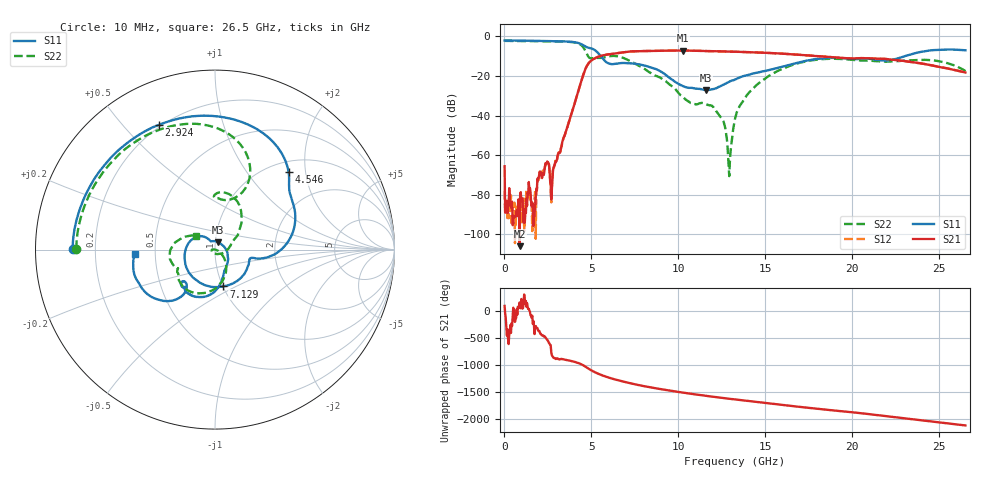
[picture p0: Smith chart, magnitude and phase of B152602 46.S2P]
!  2-Port S-parameters saved by WinCal
! VAR MeasName=S-Parameters (CALIBRATED_DATA) read from VNA (N5242A)
! VAR MeasDate=2016-1-5 16:32:47
! VAR NAME=B152602 46
! VAR FILENAME=B152602 46.S2P
! VAR DATE=2016-1-5 16:32:47
! VAR PHYS_PORTS=1,2
# Hz S DB R 50
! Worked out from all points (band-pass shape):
!   801 points, 10 MHz to 26.5 GHz, reference 50 ohm
!   highest |S21| = -7.09 dB at 10.27 GHz (marker M1); lowest = -106.1 dB at 870.9 MHz (marker M2)
!   |S21| within 3 dB of the highest: 5.439 GHz to 18.25 GHz (12.82 GHz wide, 108 % of centre)
!   lowest |S11| = -27.1 dB at 11.57 GHz (marker M3), VSWR 1.09, Z = 51.4 + j4.25 ohm
!   |S11| at or under -10 dB: 5.544 GHz to 23.01 GHz (17.46 GHz wide, 122 % of centre)
!   |S22| runs from -70.7 to -2.2 dB; largest |S21 - S12| = 0.0029
!   S11 on the Smith chart (normalised r, x): 10 MHz: 0.12, +0.00; 2.924 GHz: 0.19, +0.63; 4.546 GHz: 1.21, +1.62; 7.129 GHz: 1.00, -0.43; 26.5 GHz: 0.38, -0.02
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1e7  -2.01 179.7  -65.66 89.1  -78.01 29.6  -2.24 179.8
1.755625e8  -2.02 176.4  -89.36 16.6  -91.88 -78.4  -2.24 177.3
8.70925e8  -2.10 162.1  -106.08 152.8  -90.84 -174.8  -2.29 166.5
1.665625e9  -2.19 145.4  -95.90 169.1  -86.56 143.4  -2.35 153.9
2.427212e9  -2.29 127.6  -64.26 -161.5  -64.44 -162.1  -2.44 140.5
2.725225e9  -2.32 119.8  -77.21 -103.6  -75.45 -107.0  -2.46 134.7
2.9239e9  -2.36 114.2  -63.74 -166.0  -62.93 -165.1  -2.50 130.4
4.447075e9  -4.02 51.3  -21.76 84.5  -21.76 84.7  -4.62 74.6
4.546412e9  -4.52 46.4  -19.07 67.2  -19.07 67.3  -5.66 68.4
5.5729e9  -10.31 -7.4  -9.72 -109.2  -9.72 -109.1  -10.82 90.6
6.301375e9  -13.93 -19.1  -8.67 173.7  -8.67 173.9  -9.83 80.0
7.129188e9  -13.53 -77.3  -7.69 106.2  -7.68 106.2  -12.03 54.0
8.851038e9  -17.07 156.2  -7.26 -3.2  -7.25 -3.3  -20.37 20.1
1.027488e10  -25.13 117.9  -7.09 -75.8  -7.11 -75.8  -30.77 -59.9
1.156626e10  -27.14 69.9  -7.34 -133.6  -7.36 -133.5  -34.16 -159.3
1.252652e10  -24.69 5.8  -7.57 -173.0  -7.56 -173.0  -41.90 174.9
1.292388e10  -22.90 -14.9  -7.66 171.2  -7.65 171.4  -70.66 3.6
1.3255e10  -21.79 -28.4  -7.72 158.4  -7.71 158.5  -41.68 -18.5
1.464572e10  -18.07 -63.3  -8.12 105.2  -8.12 105.4  -23.46 -41.9
1.769208e10  -11.73 -98.3  -9.72 -4.0  -9.69 -3.8  -12.03 -104.6
2.209604e10  -12.04 -129.4  -11.54 -155.9  -11.48 -156.2  -12.71 -153.4
2.65e10  -6.97 -177.2  -18.23 37.2  -18.27 36.9  -17.54 144.4
